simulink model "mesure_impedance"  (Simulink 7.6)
settings: Solver=ode23tb  SolverMode=SingleTasking  StartTime=0.0  StopTime=0.05  RelTol=1e-4
libraries: powerlib x11

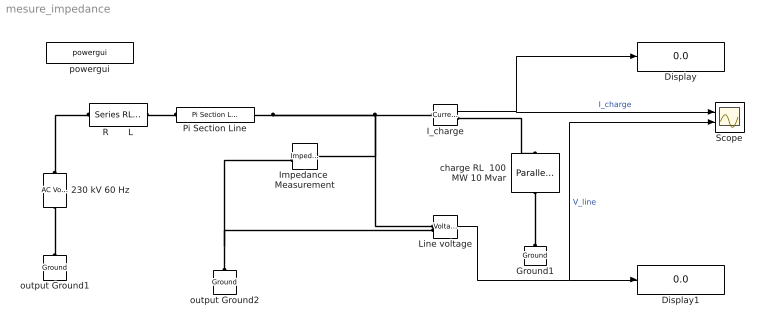
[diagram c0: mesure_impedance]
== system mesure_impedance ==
  230 kV 60 Hz : powerlib/Electrical Sources/AC Voltage Source  Description=source block  DialogController=POWERSYS.PowerSysDialog  SystemSampleTime=-1  Amplitude=230e3  Phase=0  Frequency=60  SampleTime=0  Measurements=None
  Display : Display
  Display1 : Display
  Ground1 : powerlib/Elements/Ground  DialogController=POWERSYS.PowerSysDialog  PhysicalDomain=powersysdomain  SubClassName=unknown  LeftPortType=p1  RightPortType=p1  LConnTagsString=a
  I_charge : powerlib/Measurements/Current Measurement  Tag=PoWeRsYsTeMmEaSuReMeNt  DialogController=POWERSYS.PowerSysDialog  SystemSampleTime=-1  PhasorSimulation=off  OutputType=Magnitude  PSBequivalent=0
  Impedance  Measurement : powerlib/Measurements/Impedance Measurement  DialogController=POWERSYS.PowerSysDialog  PhysicalDomain=powersysdomain  SubClassName=unknown  LeftPortType=p1  RightPortType=p1  LConnTagsString=+|-  Factor=1
  Line voltage : powerlib/Measurements/Voltage Measurement  Tag=PoWeRsYsTeMmEaSuReMeNt  DialogController=POWERSYS.PowerSysDialog  SystemSampleTime=-1  PhasorSimulation=off  OutputType=Magnitude  PSBequivalent=0
  Pi Section Line : powerlib/Elements/Pi Section Line  DialogController=POWERSYS.PowerSysDialog  PhysicalDomain=powersysdomain  SubClassName=unknown  LeftPortType=p1  RightPortType=p1  LConnTagsString=__new0  RConnTagsString=__new0  Frequency=60  Resistance=0.2568  Inductance=2e-3  Capacitance=8.6e-9  Length=100  PiSections=1  Measurements=None
  R       L : powerlib/Elements/Series RLC Branch  DialogController=POWERSYS.PowerSysDialog  PhysicalDomain=powersysdomain  SubClassName=unknown  LeftPortType=p1  RightPortType=p1  LConnTagsString=__new0  RConnTagsString=__new0  BranchType=RL  Resistance=3  Inductance=1e-2  SetiL0=off  InitialCurrent=0  Capacitance=[]  Setx0=off  InitialVoltage=0  Measurements=None
  Scope : Scope  NumInputPorts=2
  charge RL  100 MW 10 Mvar : powerlib/Elements/Parallel RLC Load  DialogController=POWERSYS.PowerSysDialog  PhysicalDomain=powersysdomain  SubClassName=unknown  LeftPortType=p1  RightPortType=p1  LConnTagsString=a  RConnTagsString=__new0  NominalVoltage=230/sqrt(2)  NominalFrequency=60  ActivePower=100e6  InductivePower=10e6  CapacitivePower=0  Setx0=off  InitialVoltage=0  SetiL0=off  InitialCurrent=0  Measurements=None
  output Ground1 : powerlib/Elements/Ground  DialogController=POWERSYS.PowerSysDialog  PhysicalDomain=powersysdomain  SubClassName=unknown  LeftPortType=p1  RightPortType=p1  LConnTagsString=a
  output Ground2 : powerlib/Elements/Ground  DialogController=POWERSYS.PowerSysDialog  PhysicalDomain=powersysdomain  SubClassName=unknown  LeftPortType=p1  RightPortType=p1  LConnTagsString=a
  powergui : powerlib/powergui  Priority=2  SystemSampleTime=-1  SimulationMode=Continuous  SampleTime=0  frequency=60  SPID=off  DisableSnubberDevices=off  DisableRonSwitches=off  DisableVfSwitches=off  SwTol=0  Interpol=off  frequencyindice=60  echomessages=off  HookPort=off  DisplayEquations=off  FunctionMessages=off  EnableUseOfTLC=off  x0status=blocks  RestoreLinks=warning  ResistiveCurrentMeasurement=off  Frange=0:200  Ylog=on  Xlog=on  ShowGrid=on  save=off  variable=ZData  ZoomFFT=on  StartTime=0.0  cycles=1  DisplayStyle=off  fundamental=60  FreqAxis=off  MaxFrequency=1000  frequencyindicesteady=1  RmsSteady=1  display=off  Ts=0  methode=off
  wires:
  Line voltage/1 -> Scope/2, Display1/1  "V_line"
  I_charge/1 -> Scope/1, Display/1  "I_charge"
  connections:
  charge RL  100 MW 10 Mvar/RConn1 -- Ground1/LConn1
  230 kV 60 Hz/RConn1 -- R       L/LConn1
  output Ground1/LConn1 -- 230 kV 60 Hz/LConn1
  Pi Section Line/RConn1 -- Impedance  Measurement/LConn1 -- I_charge/LConn1 -- Line voltage/LConn1
  I_charge/RConn1 -- charge RL  100 MW 10 Mvar/LConn1
  Pi Section Line/LConn1 -- R       L/RConn1
  output Ground2/LConn1 -- Impedance  Measurement/LConn2 -- Line voltage/LConn2
